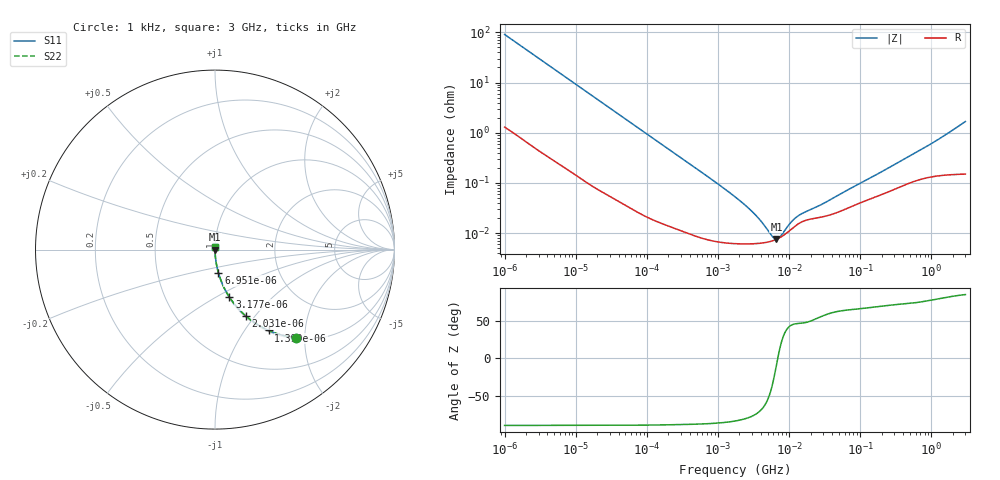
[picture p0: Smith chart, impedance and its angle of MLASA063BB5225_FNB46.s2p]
! MLASA063BB5225_FNB46  S-PARAMETER MODEL  ( Standard Model )
! Model Generated by TAIYO YUDEN Corporation (http://www.ty-top.com)
! Version 1.0
! TAIYO YUDEN Control No. 240524
! Copyright(c) 2024 TAIYO YUDEN CO.,LTD. All Rights Reserved.
! Product Description (link to TY-COMPAS)
! https://ds.yuden.co.jp/TYCOMPAS/or/detail?pn=MLASA063BB5225MFNB46&u=M
! Products Name : Multilayer Ceramic Capacitors
! Characteristics :
!  Capacitance : 2.2 [uF] , Rated Voltage : 4 [V] , TCC : X5R
!  Case Size : 0.6 x 0.3 / 0.024 x 0.012 [mm/inch] , Thickness : 0.3 / 0.012 [mm/inch]
!  (Conditions: Temperature = 25 [degC] , DC Bias Voltage = 0 [V])
! External Node Assignments :
!  1  o---| |---o  2
! GND o---------o GND
! Frequency Range : 1kHz  -  3GHz  [ 401 STEP ]
# MHZ S RI R 50
! Freq[MHz].  S11 Real  S11 Imag  S21 Real  S21 Imag  S12 Real  S12 Imag  S22 Real  S22 Imag
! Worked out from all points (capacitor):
!   401 points, 1 kHz to 3 GHz, reference 50 ohm
!   read as one part in series: C = 1.75 uF near 1.077 kHz
!   lowest |Z| = 7.64 mohm at 6.63 MHz (marker M1)
!   series resonance near 6.906 MHz, so ESL is about 300 pH
!   S11 on the Smith chart (normalised r, x): 1 kHz: 1.03, -1.81; 1.399 kHz: 1.02, -1.30; 2.031 kHz: 1.01, -0.90; 3.177 kHz: 1.01, -0.58; 6.951 kHz: 1.00, -0.27; 3 GHz: 1.00, +0.03
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0.001  0.4511 -0.4905  0.5489 0.4905  0.5489 0.4905  0.4511 -0.4905
0.001399  0.2992 -0.4507  0.7008 0.4507  0.7008 0.4507  0.2992 -0.4507
0.002031  0.1712 -0.3695  0.8288 0.3695  0.8288 0.3695  0.1712 -0.3695
0.003177  0.0799 -0.2639  0.9201 0.2639  0.9201 0.2639  0.0799 -0.2639
0.006951  0.0192 -0.1298  0.9808 0.1298  0.9808 0.1298  0.0192 -0.1298
0.01216  0.00693 -0.0756  0.9931 0.0756  0.9931 0.0756  0.00693 -0.0756
0.033275  0.00129 -0.0281  0.9987 0.0281  0.9987 0.0281  0.00129 -0.0281
0.147855  0.000205 -0.00642  0.9998 0.00642  0.9998 0.00642  0.000205 -0.00642
0.734727  7.48e-05 -0.0013  0.9999 0.0013  0.9999 0.0013  7.48e-05 -0.0013
1.732051  6.21e-05 -0.000527  0.9999 0.000527  0.9999 0.000527  6.21e-05 -0.000527
3.264662  6.18e-05 -0.000233  0.9999 0.000233  0.9999 0.000233  6.18e-05 -0.000233
5.30084  6.78e-05 -7.63e-05  0.9999 7.63e-05  0.9999 7.63e-05  6.78e-05 -7.63e-05
5.711239  6.98e-05 -5.45e-05  0.9999 5.45e-05  0.9999 5.45e-05  6.98e-05 -5.45e-05
6.629817  7.55e-05 -1.16e-05  0.9999 1.16e-05  0.9999 1.16e-05  7.55e-05 -1.16e-05
7.988506  8.72e-05 4.09e-05  0.9999 -4.09e-05  0.9999 -4.09e-05  8.72e-05 4.09e-05
10.76485  0.000121 0.000118  0.9999 -0.000118  0.9999 -0.000118  0.000121 0.000118
12.49624  0.000143 0.000148  0.9999 -0.000148  0.9999 -0.000148  0.000143 0.000148
15.05716  0.000168 0.000179  0.9998 -0.000179  0.9998 -0.000179  0.000168 0.000179
21.06097  0.000194 0.000234  0.9998 -0.000234  0.9998 -0.000234  0.000194 0.000234
256.0921  0.00068 0.00192  0.9993 -0.00192  0.9993 -0.00192  0.00068 0.00192
980.2507  0.00135 0.00582  0.9987 -0.00582  0.9987 -0.00582  0.00135 0.00582
3000  0.00178 0.0166  0.9982 -0.0166  0.9982 -0.0166  0.00178 0.0166
